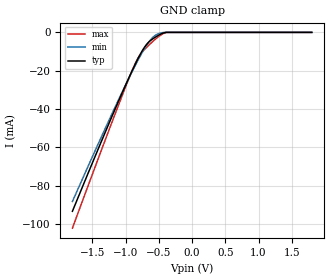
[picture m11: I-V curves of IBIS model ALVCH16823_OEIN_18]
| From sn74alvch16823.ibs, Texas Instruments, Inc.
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[Model]   ALVCH16823_OEIN_18
Model_type  Input
Vinl=0.5775
Vinh=1.2675
| variable   typ   min   max
C_comp   2.63pF   2.06pF   3.19pF
[Temperature Range]   40   100   -40
| Ambient temperature   25   85   -40
[Voltage range]   1.8   1.65   1.95
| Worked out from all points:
|   GND clamp passes 1 mA (typ) near -0.48 V on its own axis
[GND Clamp]
| ALVCH16823_OEIN_18
|   Voltage   I(typ)   I(min)   I(max)
-1.8V     -93.3mA    -88.19mA   -102.1mA
-1.235V   -46.25mA   -44.72mA   -49.56mA
-1V       -27.5mA    -27.4mA    -28.37mA
-875mV    -18.04mA   -18.61mA   -17.75mA
-795mV    -12.45mA   -13.28mA   -12.37mA
-700mV    -6.981mA   -7.539mA   -8.412mA
-615mV    -3.968mA   -3.483mA   -5.497mA
-535mV    -2.13mA    -1.195mA   -3.054mA
-445mV    -515.8uA   -125.4uA   -861.2uA
-375mV    -85.17nA   -8.524uA   -4.38uA
1.8V      24.55pA    142.2pA    23.4pA
